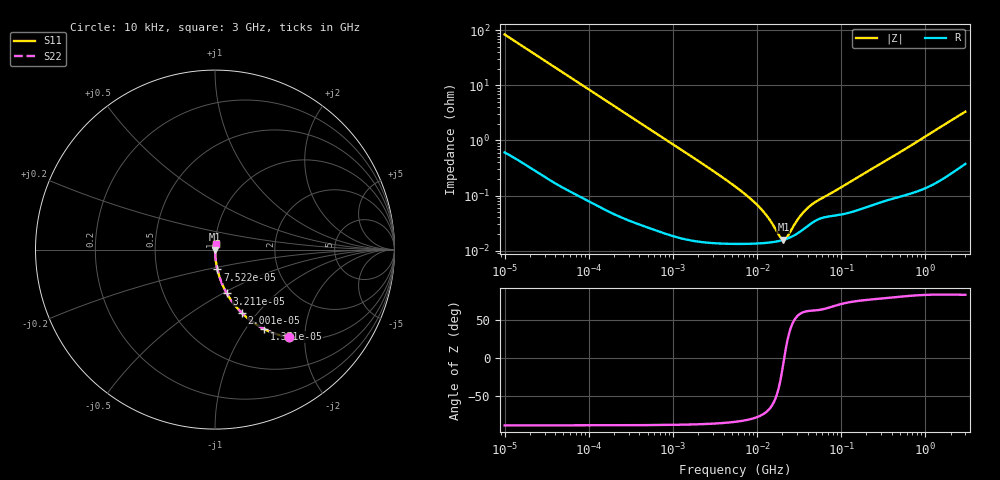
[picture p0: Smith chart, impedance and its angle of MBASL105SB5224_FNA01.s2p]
! MBASL105SB5224_FNA01  S-PARAMETER MODEL  ( Standard Model )
! Model Generated by TAIYO YUDEN Corporation (http://www.ty-top.com)
! Version 1.0
! TAIYO YUDEN Control No. 220601
! Copyright(c) 2013 TAIYO YUDEN CO.,LTD. All Rights Reserved.
! Product Description (link to TY-COMPAS)
! https://ds.yuden.co.jp/TYCOMPAS/or/detail?pn=MBASL105SB5224KFNA01&u=M
! Products Name : Multilayer Ceramic Capacitors
! Characteristics :
!  Capacitance : 0.22 [uF] , Rated Voltage : 10 [V] , TCC : X5R
!  Case Size : 1.0 x 0.5 / 0.039 x 0.02 [mm/inch] , Thickness : 0.5 / 0.02 [mm/inch]
!  (Conditions: Temperature = 25 [degC] , DC Bias Voltage = 0 [V])
! External Node Assignments :
!  1  o---| |---o  2
! GND o---------o GND
! Frequency Range : 10kHz  -  3GHz  [ 401 STEP ]
# MHZ S RI R 50
! Freq[MHz].  S11 Real  S11 Imag  S21 Real  S21 Imag  S12 Real  S12 Imag  S22 Real  S22 Imag
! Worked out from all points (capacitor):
!   401 points, 10 kHz to 3 GHz, reference 50 ohm
!   read as one part in series: C = 190 nF near 10.65 kHz
!   lowest |Z| = 15.8 mohm at 20.59 MHz (marker M1)
!   series resonance near 21.1 MHz, so ESL is about 300 pH
!   S11 on the Smith chart (normalised r, x): 10 kHz: 1.01, -1.67; 13.71 kHz: 1.01, -1.22; 20.01 kHz: 1.01, -0.84; 32.11 kHz: 1.00, -0.52; 75.22 kHz: 1.00, -0.22; 3 GHz: 1.01, +0.07
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0.01  0.4116 -0.4885  0.5884 0.4885  0.5884 0.4885  0.4116 -0.4885
0.013707  0.2731 -0.4418  0.7269 0.4418  0.7269 0.4418  0.2731 -0.4418
0.02001  0.1513 -0.3545  0.8487 0.3545  0.8487 0.3545  0.1513 -0.3545
0.03211  0.0658 -0.244  0.9342 0.244  0.9342 0.244  0.0658 -0.244
0.048377  0.0307 -0.1684  0.9693 0.1684  0.9693 0.1684  0.0307 -0.1684
0.075221  0.0134 -0.1105  0.9866 0.1105  0.9866 0.1105  0.0134 -0.1105
0.082683  0.0112 -0.1008  0.9888 0.1008  0.9888 0.1008  0.0112 -0.1008
0.199902  0.00225 -0.0423  0.9977 0.0423  0.9977 0.0423  0.00225 -0.0423
0.683653  0.000378 -0.0125  0.9996 0.0125  0.9996 0.0125  0.000378 -0.0125
2.652321  0.000149 -0.00318  0.9999 0.00318  0.9999 0.00318  0.000149 -0.00318
5.477226  0.000135 -0.00146  0.9999 0.00146  0.9999 0.00146  0.000135 -0.00146
8.252149  0.000134 -0.000883  0.9999 0.000883  0.9999 0.000883  0.000134 -0.000883
10.95979  0.000136 -0.000574  0.9999 0.000574  0.9999 0.000574  0.000136 -0.000574
14.10408  0.000141 -0.000339  0.9999 0.000339  0.9999 0.000339  0.000141 -0.000339
18.73182  0.000151 -9.78e-05  0.9998 9.78e-05  0.9998 9.78e-05  0.000151 -9.78e-05
20.5901  0.000157 -2e-05  0.9998 2e-05  0.9998 2e-05  0.000157 -2e-05
22.63272  0.000165 5.75e-05  0.9998 -5.75e-05  0.9998 -5.75e-05  0.000165 5.75e-05
29.12589  0.000198 0.000266  0.9998 -0.000266  0.9998 -0.000266  0.000198 0.000266
34.09912  0.000233 0.000397  0.9998 -0.000397  0.9998 -0.000397  0.000233 0.000397
45.28751  0.000321 0.000617  0.9997 -0.000617  0.9997 -0.000617  0.000321 0.000617
374.4521  0.000861 0.0046  0.9991 -0.0046  0.9991 -0.0046  0.000861 0.0046
3000  0.00482 0.0327  0.9952 -0.0327  0.9952 -0.0327  0.00482 0.0327
